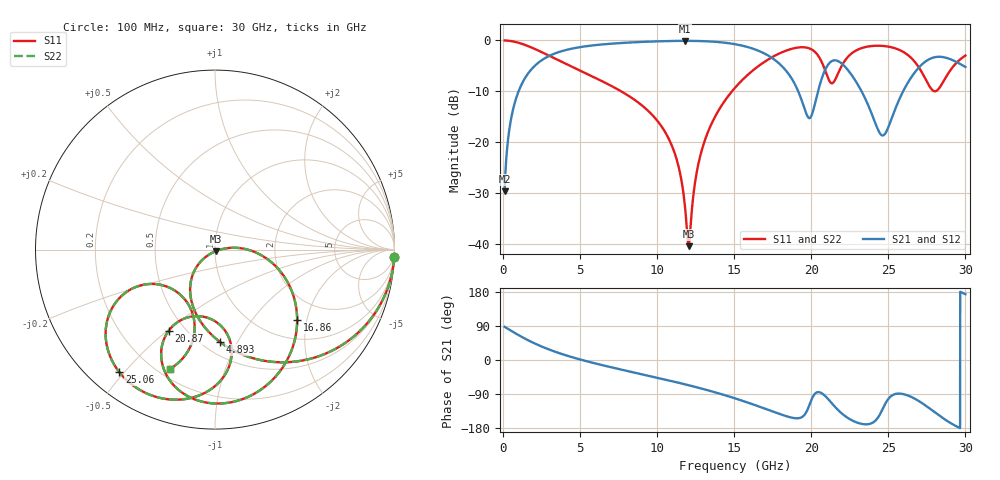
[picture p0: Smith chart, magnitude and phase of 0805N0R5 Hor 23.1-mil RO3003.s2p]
# GHz S MA R 50
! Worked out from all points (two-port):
!   3201 points, 100 MHz to 30 GHz, reference 50 ohm
!   highest |S21| = -0.09 dB at 11.83 GHz (marker M1); lowest = -29.6 dB at 100 MHz (marker M2)
!   |S21| within 3 dB of the highest: 2.964 GHz to 17.27 GHz (14.3 GHz wide, 141 % of centre)
!   lowest |S11| = -40.4 dB at 12.04 GHz (marker M3), VSWR 1.02, Z = 50.4 - j0.891 ohm
!   |S11| at or under -10 dB: 7.667 GHz to 14.85 GHz (7.185 GHz wide, 63.8 % of centre)
!   |S22| runs from -40.4 to 0.0 dB; largest |S21 - S12| = 0
!   S11 on the Smith chart (normalised r, x): 100 MHz: 1, -46; 4.893 GHz: 0.61, -0.85; 16.86 GHz: 1.43, -1.75; 20.87 GHz: 0.41, -0.51; 25.06 GHz: 0.09, -0.48; 30 GHz: 0.25, -0.66
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0.1  0.9994 -2.5  0.03315 87.5  0.03315 87.5  0.9994 -2.5
0.5485  0.9838 -13.5  0.179 76.5  0.179 76.5  0.9838 -13.5
1.342719  0.9131 -31.9  0.4067 58.1  0.4067 58.1  0.9131 -31.9
4.893344  0.5141 -87.1  0.8544 2.6  0.8544 2.6  0.5141 -87.1
5.089563  0.4976 -89.2  0.8639 0.4  0.8639 0.4  0.4976 -89.2
10.06978  0.1584 -135.0  0.9803 -47.4  0.9803 -47.4  0.1584 -135.0
11.22841  0.07082 -141.8  0.9889 -58.4  0.9889 -58.4  0.07082 -141.8
11.82641  0.02159 -129.3  0.9902 -64.4  0.9902 -64.4  0.02159 -129.3
12.04131  0.009552 -67.8  0.99 -66.6  0.99 -66.6  0.009552 -67.8
13.00372  0.09496 6.2  0.9834 -76.7  0.9834 -76.7  0.09496 6.2
15.05  0.343 -14.6  0.9187 -101.2  0.9187 -101.2  0.343 -14.6
16.86269  0.6019 -40.5  0.7567 -126.4  0.7567 -126.4  0.6019 -40.5
18.937  0.8419 -77.6  0.3712 -153.5  0.3712 -153.5  0.8419 -77.6
20.03956  0.8127 -103.8  0.1867 -102.3  0.1867 -102.3  0.8127 -103.8
20.87116  0.522 -119.8  0.5036 -93.8  0.5036 -93.8  0.522 -119.8
22.15125  0.6235 -81.9  0.5599 -146.7  0.5599 -146.7  0.6235 -81.9
23.422  0.8543 -102.3  0.284 -169.5  0.284 -169.5  0.8543 -102.3
25.01978  0.8683 -127.4  0.1432 -101.7  0.1432 -101.7  0.8683 -127.4
25.05716  0.8662 -128.0  0.1481 -99.9  0.1481 -99.9  0.8662 -128.0
27.46784  0.4029 -151.7  0.6297 -121.7  0.6297 -121.7  0.4029 -151.7
28.63581  0.4109 -106.4  0.6823 -155.9  0.6823 -155.9  0.4109 -106.4
30  0.7105 -110.6  0.5486 173.7  0.5486 173.7  0.7105 -110.6
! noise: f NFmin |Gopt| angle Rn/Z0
0.1  0.001671  0.9715  1.553  0.01332
3.417  0.007676  0.7538  21.97  0.006071
6.743  0.0131  0.724  39.93  0.008352
10.06  0.01934  0.7287  56.94  0.01104
13.39  0.02998  0.7703  72.93  0.01737
16.7  0.06431  0.8646  88.35  0.05271
20.03  0.645  0.9832  103.5  3.385
23.35  0.3384  0.9641  117.1  0.5811
26.67  0.3179  0.9571  130.3  0.2953
30  0.2081  0.9282  142.6  0.06698
